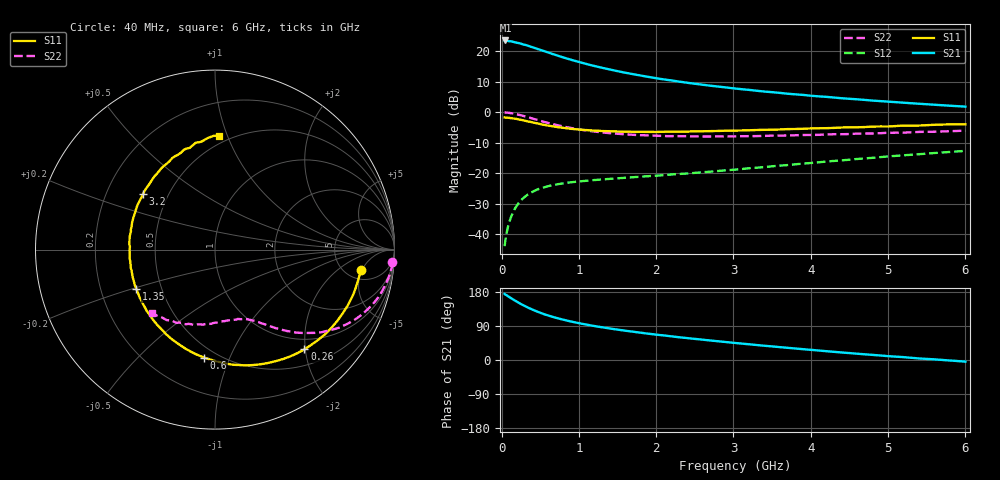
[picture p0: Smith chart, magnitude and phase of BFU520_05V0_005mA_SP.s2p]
! Filename:  P:\Prog\Test\Noise\ATS_data\Testdata_Net\03 Spar\BFU520_APG2013_37_A05_05p0V_005mA_SP_CM01_D.s2p
! Date/Time: Fri 26/Apr/2013 13:00:08
! BFU520_APG2013_37_A05_05p0V_1to20mA_SP_CM01_Bias4_R.s2p
! MDIF S-parameter v. bias file
! BFU520_APG2013_37_A05_05p0V_1to20mA_SP_CM01
! Date/time Tue Apr 23 15:26:19 2013
! VAR V_out= 5.0000
! VAR I_out= 5.0000
! VAR V_in= 0.8272
! VAR I_in= 0.0564
! Device data file deembeded for feedlines and parallel
! Original file: \03 Spar\BFU520_APG2013_37_A05_05p0V_005mA_SP_CM01_R.s2p
! Feed-files: PR047V01_250413_Feed1.s2p, PR047V01_250413_Feed2.s2p
! Parallel-file: PR047V01_250413_Par.s2p
# MHz S MA R 50
!  Freq-MHz  S11-mag  S11-arg  S21-mag  S21-arg  S12-mag  S12-arg  S22-mag  S22-arg
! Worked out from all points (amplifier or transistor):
!   98 points, 40 MHz to 6 GHz, reference 50 ohm
!   highest |S21| = 23.5 dB at 50 MHz (marker M1)
!   |S21| within 3 dB of that: start of sweep to 491.6 MHz
!   unconditionally stable (mu >= 1): 2.294 GHz to 4.411 GHz
!   at 300 MHz: K = 0.19, MSG = 24.9 dB, |S12| = -27.7 dB
!   at 1.6 GHz: K = 0.82, MSG = 17.2 dB, |S12| = -21.4 dB
!   at 6 GHz: K = 0.85, MSG = 7.2 dB, |S12| = -12.6 dB
!   S11 on the Smith chart (normalised r, x): 40 MHz: 6.88, -4.70; 260 MHz: 0.79, -1.98; 600 MHz: 0.43, -0.81; 1.35 GHz: 0.36, -0.21; 3.2 GHz: 0.36, +0.30; 6 GHz: 0.44, +0.94
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40  0.8204 -7.8  14.91 174.3  0.006439 85.5  0.9914 -4.1
50  0.8182 -9.7  14.93 172.4  0.00802 84.5  0.9902 -5.2
70  0.8141 -13.4  14.72 170.4  0.01122 82.7  0.985 -7.3
140  0.7947 -26.9  14.29 161.0  0.02174 75.7  0.9576 -14.4
220  0.7635 -41.3  13.57 151.3  0.03238 68.5  0.9111 -21.6
260  0.7463 -48.1  13.12 146.8  0.03702 65.3  0.8857 -24.9
320  0.7182 -58.0  12.5 140.5  0.04315 60.9  0.844 -29.5
400  0.6826 -70.0  11.56 132.9  0.04981 56.1  0.7882 -34.5
500  0.6411 -83.6  10.48 124.8  0.05659 51.1  0.7256 -39.7
600  0.6049 -95.7  9.524 117.7  0.06154 47.4  0.6698 -43.9
700  0.5773 -106.1  8.632 111.6  0.06542 44.5  0.6229 -47.2
800  0.5547 -115.5  7.869 106.3  0.06871 42.5  0.5836 -50.0
1050  0.5143 -135.2  6.388 95.2  0.07466 39.4  0.5124 -55.5
1350  0.4902 -153.3  5.161 84.8  0.08032 38.2  0.4605 -60.2
1600  0.4794 -166.0  4.431 77.3  0.08463 38.1  0.4349 -64.0
2050  0.4779 176.5  3.515 65.9  0.09233 39.4  0.4104 -70.5
2450  0.4848 162.6  2.974 56.7  0.1003 40.8  0.4015 -76.8
3100  0.5026 144.3  2.384 43.5  0.1176 43.2  0.4044 -86.6
3200  0.5064 142.5  2.321 41.5  0.1211 43.4  0.4063 -88.0
4100  0.5468 121.1  1.818 25.1  0.1514 43.4  0.4268 -102.9
5200  0.6048 100.3  1.431 7.5  0.1974 39.5  0.4632 -121.3
6000  0.6355 87.8  1.235 -4.3  0.2331 34.4  0.4985 -134.8
